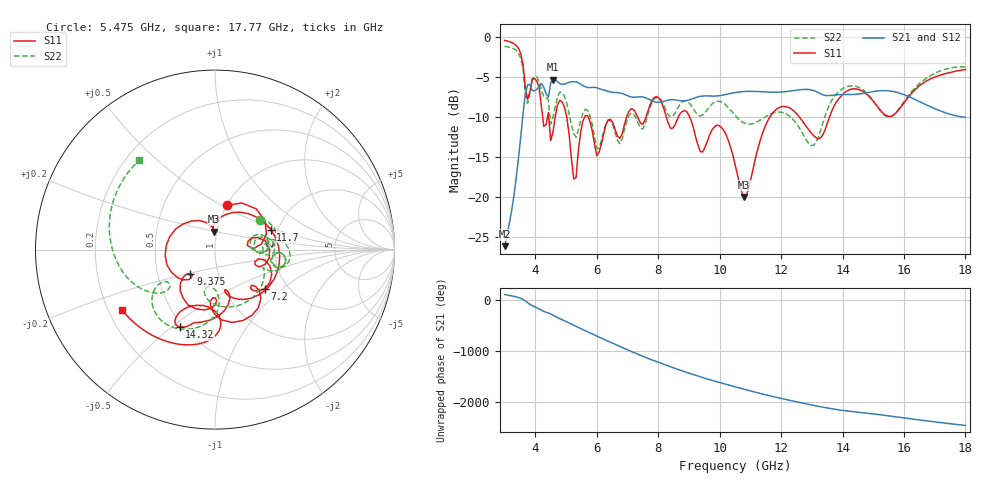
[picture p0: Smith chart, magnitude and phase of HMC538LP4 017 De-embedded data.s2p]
! Chelmsford, MA 01824
! http://www.hittite.com
! Tel: 978-250-3343
! Fax: 978-250-3373
! Device  :  HMC538LP4
! Description:  600 Analog Phase Shifter
! Frequency  :  6.0 GHz - 15.0 GHz
! Package  :  LP4  - 4x4 mm Quad Flatpack No-Lead (QFN) Plastic Package: 24 pin
! Ports  :  2 RF, 1 DC
!  Pin  3  = Rfin  = Port 1
!  Pin  16  = Rfout = Port 2
!  pin  21  = vCTL
! Voltages:  VCTL  = 0 to 5.0 Volts
! Currents :  Vb(V)  Vd(V)  Ib(mA)  Id(mA)
!  0.00  1.70  0.000000	0.485044
! Data:  The device was measured on evaluation board 111296-1.
!  Data was collected using a calibrated network analyzer.
!  The evaluation circuit board was modeled and simulated.This was use
!  to removed the evaluation board circuit from the measured data.
!  The reference plane is the center of the package pin.
! Misc:  Lot #
!Date Measured:  03 - 11 -2009
! Date:  03 - 17 -2009
! Note:
!  Hittite Microwave supplies this data as a sample of measured data at the
!  package pin for this package product.  Your particular data for this product
!  may vary.
!  Data was taken at 25 degrees C.
!  Hittite Microwave reserves the right to change this data at anytime.
# MHz S MA R 50
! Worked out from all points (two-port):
!   201 points, 3 GHz to 18 GHz, reference 50 ohm
!   highest |S21| = -5.30 dB at 4.575 GHz (marker M1); lowest = -26.2 dB at 3 GHz (marker M2)
!   |S21| within 3 dB of the highest: 3.639 GHz to 16.63 GHz (12.99 GHz wide, 128 % of centre)
!   lowest |S11| = -20.0 dB at 10.8 GHz (marker M3), VSWR 1.22, Z = 48.3 + j9.68 ohm
!   |S11| at or under -10 dB: 5.718 GHz to 6.971 GHz (1.253 GHz wide, 19.7 % of centre); 9.023 GHz to 11.63 GHz (2.612 GHz wide, 25.3 % of centre); 12.6 GHz to 13.57 GHz (979.6 MHz wide, 7.49 % of centre)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
!   |S22| runs from -13.9 to -1.1 dB; largest |S21 - S12| = 0.0011
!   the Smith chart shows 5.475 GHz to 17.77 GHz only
!   S11 on the Smith chart (normalised r, x): 5.475 GHz: 1.00, +0.53; 7.2 GHz: 1.53, -0.76; 9.375 GHz: 0.74, -0.21; 11.7 GHz: 1.83, +0.46; 14.32 GHz: 0.48, -0.53; 17.77 GHz: 0.26, -0.28
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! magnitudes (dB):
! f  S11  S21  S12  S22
! 3 GHz  -0.4  -26.2  -26.2  -1.1
! 3.525 GHz  -2.0  -12.5  -12.5  -2.6
! 3.75 GHz  -7.8  -6.0  -6.0  -8.3
! 4.05 GHz  -5.5  -6.5  -6.5  -5.0
! 4.575 GHz  -11.9  -5.3  -5.3  -10.0
! 4.875 GHz  -8.1  -5.9  -5.9  -7.0
! 5.25 GHz  -17.8  -5.6  -5.6  -12.1
! 5.475 GHz  -11.9  -5.9  -5.9  -10.4
! 5.55 GHz  -10.5  -6.1  -6.1  -9.5
! 6 GHz  -14.8  -6.3  -6.3  -13.9
! 7.2 GHz  -9.1  -7.5  -7.5  -9.6
! 8.025 GHz  -7.6  -8.2  -8.2  -7.6
! 9.375 GHz  -14.3  -7.4  -7.4  -9.8
! 9.975 GHz  -11.1  -7.3  -7.3  -8.0
! 10.5 GHz  -15.9  -6.9  -6.9  -9.8
! 10.8 GHz  -20.0  -6.8  -6.8  -10.7
! 11.7 GHz  -9.6  -6.9  -6.9  -9.5
! 13.05 GHz  -12.3  -6.7  -6.7  -13.6
! 14.32 GHz  -6.5  -7.2  -7.2  -6.1
! 15.53 GHz  -9.9  -6.7  -6.7  -10.0
! 17.77 GHz  -4.2  -9.9  -9.9  -3.7
! 18 GHz  -4.0  -10.0  -10.0  -3.7
